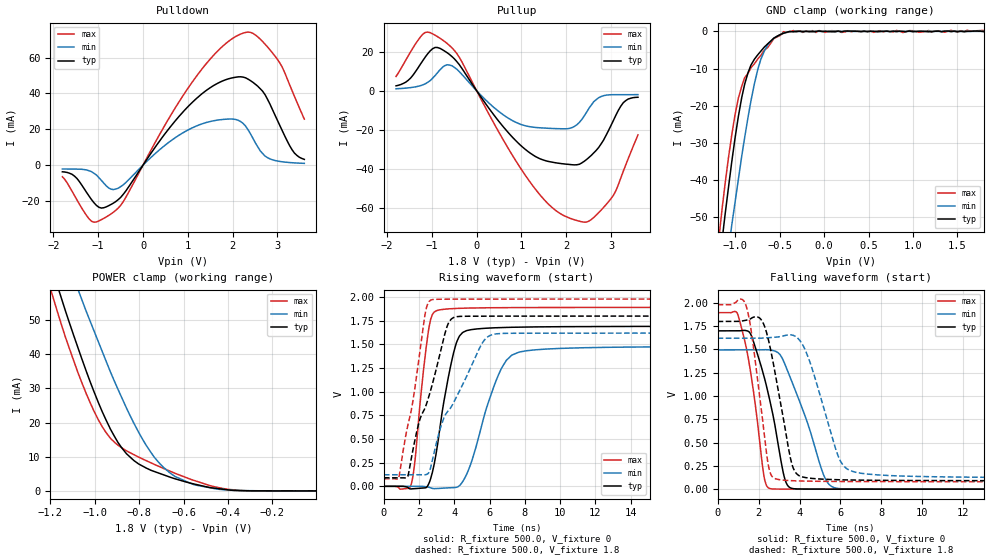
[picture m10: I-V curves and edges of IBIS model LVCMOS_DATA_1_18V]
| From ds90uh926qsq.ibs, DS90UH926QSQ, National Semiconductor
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[Model] LVCMOS_DATA_1_18V
Model_type 3-state
Enable Active-High
Vmeas = 0.9V
Cref = 0.0pF
Rref = 1.0e10
Vref = 0.0V
C_comp   3.52pF   2.88pF   4.05pF
[Voltage Range]   1.8V   1.62V   1.98V
[Temperature Range]   25.0   130.0   -40.0
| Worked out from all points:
|   slope of the pulldown table from 0 to 0.27 V, typ, clamps not added: 27.1 ohm
|   slope of the pullup table from 0 to 0.27 V, typ, clamps not added: 30.4 ohm
|   GND clamp passes 1 mA (typ) near -0.51 V on its own axis
|   POWER clamp passes 1 mA (typ) near -0.48 V on its own axis
|   rising waveform, R_fixture 500.0, V_fixture 0: 20-80 % time 927ps typ, 1.49ns min, 609ps max; typ from 0 V to 1.69 V
|   falling waveform, R_fixture 500.0, V_fixture 0: 20-80 % time 992ps typ, 1.4ns min, 719ps max; typ from 1.7 V to 0 V
|   rising waveform, R_fixture 500.0, V_fixture 1.8: 20-80 % time 1.56ns typ, 2.15ns min, 999ps max; typ from 0.09 V to 1.8 V
|   falling waveform, R_fixture 500.0, V_fixture 1.8: 20-80 % time 842ps typ, 1.2ns min, 640ps max; typ from 1.8 V to 0.09 V
[GND Clamp]
-1.8V     -200.3mA   -195.1mA   -211.1mA
-1.186V   -63.69mA   -78.16mA   -55.71mA
-1.148V   -55.71mA   -71.1mA    -47.34mA
-1.115V   -49.06mA   -65.26mA   -40.78mA
-1.038V   -34.6mA    -51.66mA   -27.43mA
-966.7mV  -22.93mA   -39.86mA   -18mA
-895.4mV  -14.21mA   -28.56mA   -12.45mA
-824.2mV  -9.037mA   -18.62mA   -9.755mA
-747.4mV  -6.277mA   -10.23mA   -7.411mA
-637.8mV  -3.38mA    -3.686mA   -4.378mA
-456.9mV  -497.9uA   -465.5uA   -69.16uA
1.796V    -65.2uA    0A         234.3uA
[POWER Clamp]
-1.8V     198.7mA    195mA      208.6mA
-1.186V   63.72mA    78.5mA     56.28mA
-1.148V   55.89mA    71.56mA    48.16mA
-1.06V    38.99mA    56.29mA    31.98mA
-966.7mV  23.26mA    40.88mA    18.84mA
-928.3mV  17.96mA    34.67mA    15.32mA
-879mV    12.65mA    27.39mA    12.64mA
-769.3mV  6.72mA     13.44mA    8.883mA
-659.7mV  3.988mA    5.182mA    5.735mA
-550.1mV  1.973mA    1.753mA    2.998mA
-402mV    324.7uA    275.7uA    472.1uA
-1.827mV  -2.938uA   -12.37uA   -3.12uA
[Pullup]
-1.8V     2.538mA    1.037mA    7.355mA
-1.148V   17.33mA    3.544mA    29.96mA
-714.5mV  20.36mA    12.9mA     25.27mA
-385.6mV  13.35mA    9.771mA    17.08mA
431.3mV   -13.83mA   -9.445mA   -18.61mA
1.089V    -30.12mA   -17.96mA   -43.47mA
1.742V    -36.84mA   -19.37mA   -60.98mA
2.345V    -37.01mA   -14.77mA   -67.18mA
2.668V    -30.55mA   -4.519mA   -63.78mA
3.052V    -15.2mA    -1.996mA   -53.57mA
3.271V    -6.135mA   -1.984mA   -41.35mA
3.6V      -3.31mA    -1.967mA   -22.59mA
[Pulldown]
-1.8V     -3.706mA   -2.144mA   -6.494mA
-1.477V   -7.386mA   -2.221mA   -19.29mA
-1.148V   -19.3mA    -3.654mA   -31.36mA
-928.3mV  -23.95mA   -8.523mA   -30.41mA
-659.7mV  -21.18mA   -13.63mA   -26.23mA
1.144V    36.08mA    21.32mA    47.92mA
1.961V    48.53mA    25.76mA    70.06mA
2.29V     48.72mA    21.76mA    74.07mA
2.668V    41.3mA     6.545mA    69.01mA
3.052V    22.22mA    2.074mA    57.1mA
3.381V    6.694mA    1.265mA    38.33mA
3.6V      3.213mA    998.2uA    25.68mA
[Rising Waveform]
R_fixture=500.0
V_fixture=0
V_fixture_min=0
V_fixture_max=0
0s        22.28nV    566.7nV    3.79nV
1.55ns    -27.62mV   259.4nV    22.3mV
2.55ns    29.98mV    -9.55mV    1.675V
3.15ns    581mV      -21.6mV    1.866V
3.8ns     1.288V     -14.93mV   1.878V
4.3ns     1.593V     9.477mV    1.882V
4.9ns     1.655V     223.3mV    1.885V
6.65ns    1.679V     1.241V     1.889V
8.05ns    1.684V     1.433V     1.89V
49.98ns   1.694V     1.484V     1.893V
[Falling Waveform]
R_fixture=500.0
V_fixture=0
V_fixture_min=0
V_fixture_max=0
0s        1.699V     1.495V     1.895V
1ns       1.699V     1.495V     1.866V
1.65ns    1.647V     1.495V     1.203V
2.25ns    1.224V     1.497V     158.4mV
2.6ns     903.4mV    1.493V     4.399mV
3.2ns     183.3mV    1.385V     733.1uV
3.45ns    31.98mV    1.253V     582.3uV
5.2ns     506.5uV    140.7mV    217.5uV
5.9ns     361.5uV    6.865mV    166.1uV
49.98ns   5.796uV    14.75uV    3.591uV
[Rising Waveform]
R_fixture=500.0
V_fixture=1.8
V_fixture_min=1.62
V_fixture_max=1.98
0s        90.38mV    122.1mV    79.85mV
850ps     90.38mV    122.1mV    96.53mV
1.35ns    104.1mV    122.1mV    639.9mV
1.95ns    648.5mV    122.1mV    1.302V
2.35ns    836.9mV    122.3mV    1.835V
2.75ns    1.082V     280mV      1.975V
3.8ns     1.764V     833.7mV    1.979V
5.55ns    1.799V     1.506V     1.98V
6.3ns     1.799V     1.61V      1.98V
49.98ns   1.8V       1.62V      1.98V
[Falling Waveform]
R_fixture=500.0
V_fixture=1.8
V_fixture_min=1.62
V_fixture_max=1.98
0s        1.8V       1.62V      1.98V
1.4ns     1.813V     1.62V      1.963V
2.05ns    1.838V     1.62V      1.004V
2.45ns    1.632V     1.625V     290.9mV
3ns       1.012V     1.635V     102.4mV
3.85ns    167.3mV    1.632V     89.03mV
4.5ns     117.8mV    1.37V      85.53mV
5.95ns    100.8mV    323.6mV    82.45mV
6.95ns    96.83mV    172.3mV    81.48mV
49.98ns   90.38mV    122.1mV    79.85mV
[Ramp]
R_load = 500.0
dV/dt_r   1.016287E0/9E-10   8.905728E-1/1.5E-9   1.135646E0/6E-10
dV/dt_f   1.02577E0/8.5E-10   8.987482E-1/1.2E-9   1.140088E0/6E-10
